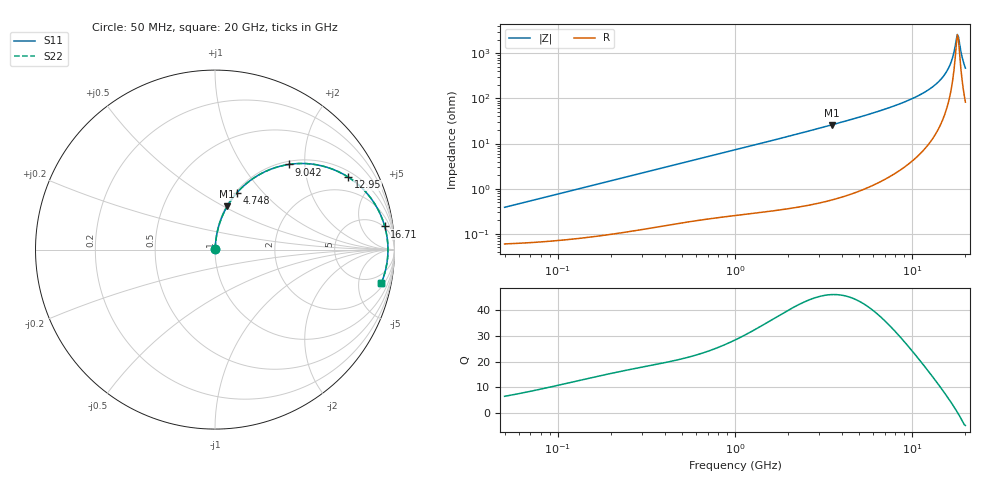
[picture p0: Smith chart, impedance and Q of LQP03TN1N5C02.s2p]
!Murata Part Number: LQP03TN1N5C02
!These Parameters are Measured in Series Mode Connection
!  o--[Z]--o
!Port1  Port2
!  o-------o
!Freq. Start=50[MHz] Stop=20[GHz], 401[Steps]
# Hz S RI R 50
!Freq.(Hz) S11(Real) S11(Imag) S21(Real) S21(Imag) S12(Real) S12(Imag) S22(Real) S22(Imag)
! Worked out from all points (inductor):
!   401 points, 50 MHz to 20 GHz, reference 50 ohm
!   read as one part in series: L = 1.22 nH near 51.52 MHz
!   highest Q = 46.2 at 3.519 GHz (marker M1), where L = 1.18 nH
!   self-resonance near 18.01 GHz
!   S11 on the Smith chart (normalised r, x): 50 MHz: 1.00, +0.01; 4.748 GHz: 1.02, +0.72; 9.042 GHz: 1.06, +1.67; 12.95 GHz: 1.24, +3.52; 16.71 GHz: 5, +13; 20 GHz: 2.66, -9.28
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5e7  0.000613 0.00383  0.9994 -0.00383  0.9994 -0.00383  0.000613 0.00383
1.364002e8  0.000912 0.0103  0.9991 -0.0103  0.9991 -0.0103  0.000912 0.0103
3.721004e8  0.00219 0.0274  0.9978 -0.0274  0.9978 -0.0274  0.00219 0.0274
1e9  0.00772 0.0717  0.9923 -0.0717  0.9923 -0.0717  0.00772 0.0717
2.728004e9  0.042 0.1896  0.958 -0.1896  0.958 -0.1896  0.042 0.1896
3.519108e9  0.0678 0.2408  0.9322 -0.2408  0.9322 -0.2408  0.0678 0.2408
4.748272e9  0.1206 0.3146  0.8794 -0.3146  0.8794 -0.3146  0.1206 0.3146
6.034176e9  0.1919 0.3814  0.8081 -0.3814  0.8081 -0.3814  0.1919 0.3814
7.442007e9  0.287 0.438  0.713 -0.438  0.713 -0.438  0.287 0.438
9.041845e9  0.4128 0.4746  0.5872 -0.4746  0.5872 -0.4746  0.4128 0.4746
1.098561e10  0.5792 0.4701  0.4208 -0.4701  0.4208 -0.4701  0.5792 0.4701
1.295331e10  0.7421 0.4041  0.2579 -0.4041  0.2579 -0.4041  0.7421 0.4041
1.396067e10  0.8149 0.3469  0.1851 -0.3469  0.1851 -0.3469  0.8149 0.3469
1.504638e10  0.8801 0.2701  0.1199 -0.2701  0.1199 -0.2701  0.8801 0.2701
1.597544e10  0.9224 0.194  0.0776 -0.194  0.0776 -0.194  0.9224 0.194
1.670968e10  0.9459 0.1288  0.0541 -0.1288  0.0541 -0.1288  0.9459 0.1288
1.774144e10  0.9626 0.0321  0.0374 -0.0321  0.0374 -0.0321  0.9626 0.0321
1.800918e10  0.9637 0.00639  0.0363 -0.00639  0.0363 -0.00639  0.9637 0.00639
1.828096e10  0.9634 -0.0199  0.0366 0.0199  0.0366 0.0199  0.9634 -0.0199
1.855685e10  0.9616 -0.0467  0.0384 0.0467  0.0384 0.0467  0.9616 -0.0467
1.940974e10  0.9462 -0.1296  0.0538 0.1296  0.0538 0.1296  0.9462 -0.1296
2e10  0.9264 -0.1866  0.0736 0.1866  0.0736 0.1866  0.9264 -0.1866
